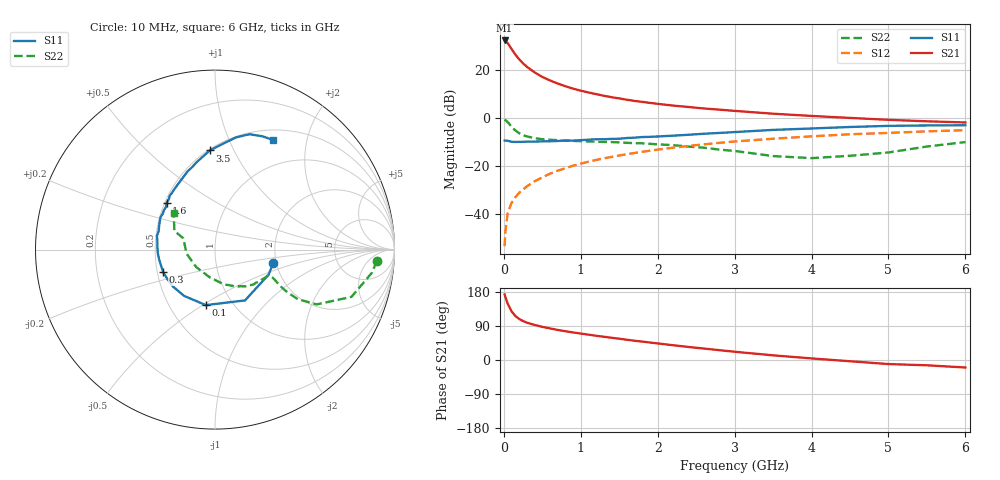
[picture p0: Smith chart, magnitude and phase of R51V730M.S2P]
! SIEMENS Small Signal Semiconductors
! BFR183
! Si NPN RF Bipolar Junction Transistor in SOT23
! VCE = 1.75 V  IC = 30 mA
! Common Emitter S-Parameters:  May  1996
# GHz  S  MA  R  50
!  f  S11  S21  S12  S22
! GHz  MAG  ANG  MAG  ANG  MAG  ANG  MAG  ANG
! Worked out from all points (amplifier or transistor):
!   36 points, 10 MHz to 6 GHz, reference 50 ohm
!   highest |S21| = 32.1 dB at 10 MHz (marker M1)
!   |S21| within 3 dB of that: start of sweep to 88.78 MHz
!   unconditionally stable (mu >= 1): start of sweep to 10.02415 MHz; 339.5 MHz to 2.541 GHz
!   at 250 MHz: K = 0.95, MSG = 26.2 dB, |S12| = -30.0 dB
!   at 1.4 GHz: K = 1.08, MAG = 10.7 dB, |S12| = -16.4 dB
!   at 6 GHz: K = 0.94, MSG = 1.6 dB, |S12| = -5.3 dB
!   S11 on the Smith chart (normalised r, x): 10 MHz: 1.92, -0.33; 100 MHz: 0.75, -0.52; 300 MHz: 0.54, -0.15; 1.6 GHz: 0.51, +0.31; 3.5 GHz: 0.51, +0.81; 6 GHz: 0.63, +1.47
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0.01  0.3329 -13.4  40.24 173.1  0.0021 80.0  0.904 -3.9
0.02  0.3297 -25.0  39.53 166.3  0.0042 83.7  0.8837 -8.4
0.05  0.3289 -59.4  35.43 148.7  0.0102 72.8  0.8047 -19.1
0.1  0.3135 -99.4  26.74 128.6  0.0167 70.0  0.644 -28.3
0.15  0.3102 -123.7  20.43 116.0  0.022 68.1  0.5376 -30.9
0.2  0.3117 -138.4  16.27 108.2  0.0272 69.2  0.4715 -30.6
0.25  0.3118 -148.6  13.39 102.7  0.0318 69.8  0.4294 -29.6
0.3  0.3152 -156.4  11.38 98.6  0.037 71.2  0.4048 -28.6
0.4  0.3157 -169.1  8.704 92.5  0.0471 72.7  0.3727 -26.8
0.5  0.3192 -175.9  7.01 87.4  0.0568 73.4  0.3536 -25.8
0.6  0.3213 177.3  5.911 83.3  0.0677 73.1  0.3448 -25.5
0.7  0.3251 171.1  5.108 79.4  0.0781 72.9  0.338 -25.9
0.8  0.3325 166.6  4.482 76.0  0.088 72.2  0.3313 -26.4
0.9  0.3304 161.7  3.993 72.7  0.0994 71.6  0.3259 -27.1
1.1  0.3454 152.9  3.324 66.9  0.1204 70.2  0.3183 -29.8
1.3  0.353 145.6  2.839 61.3  0.1414 68.0  0.3106 -32.4
1.6  0.3752 136.0  2.346 53.4  0.1726 64.7  0.2977 -37.7
2.2  0.4193 119.4  1.772 39.0  0.2356 57.7  0.2661 -50.3
3.5  0.5532 93.0  1.202 12.3  0.3623 39.9  0.1577 -100.5
4.5  0.6357 79.4  0.982 -3.3  0.4489 26.3  0.1599 -171.7
5.5  0.6841 67.4  0.835 -14.0  0.5158 14.1  0.2492 155.3
6  0.6911 62.2  0.789 -19.8  0.5456 6.4  0.3085 138.2
